FUNCTION "ROBOT_INRFACE" : VOID
TITLE =BLOCK ROBOT 1 AND 2 INTERFACE
AUTHOR : Esposito
FAMILY : EGAL_srl
NAME : ROB_INT
VERSION : 0.1


VAR_TEMP
  Tem_Cycle1_1 : BOOL ;
  Tem_cycle2_1 : BOOL ;
  Tem_cycle3_1 : BOOL ;
  Tem_cycle1_2 : BOOL ;
  Tem_cycle2_2 : BOOL ;
  Tem_cycle3_2 : BOOL ;
  Cycle_R1 : BOOL ;
  Cycle_R2 : BOOL ;
  Reserve : BYTE ;
  Reserve1 : INT ;
  Reserve2 : INT ;
  Reserve3 : INT ;
  Reserve4 : INT ;
  Rob1_Cycle : INT ;
  Rob2_Cycle : INT ;
END_VAR
BEGIN
NETWORK
TITLE =RESET ROBOT 1 AND 2 - rdiResetNood1 - rdiResetNood2
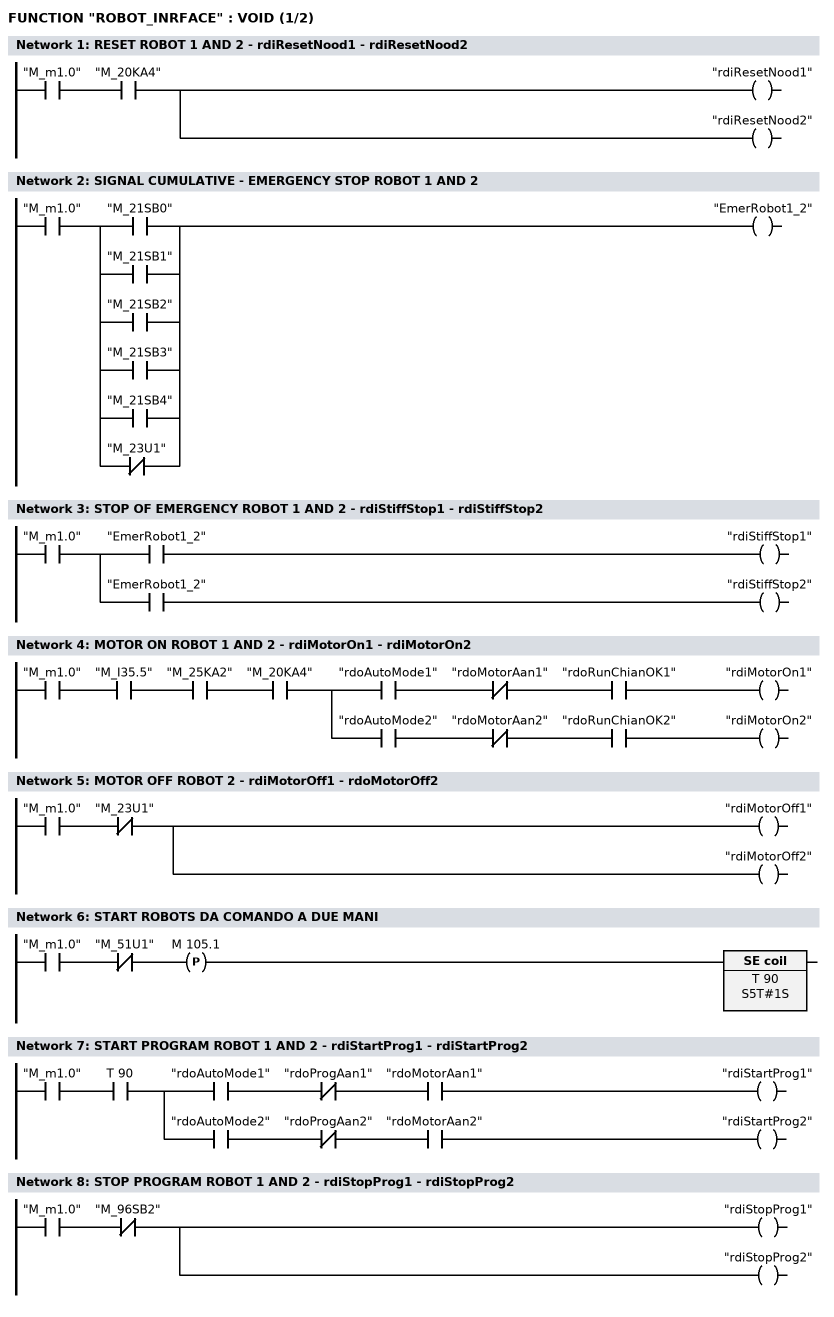
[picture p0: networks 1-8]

      U     "M_m1.0";
      U     "M_20KA4";
      =     "rdiResetNood1";
      =     "rdiResetNood2";
NETWORK
TITLE =SIGNAL CUMULATIVE - EMERGENCY STOP ROBOT 1 AND 2

      U     "M_m1.0";
      U(    ;
      O     "M_21SB0";
      O     "M_21SB1";
      O     "M_21SB2";
      O     "M_21SB3";
      O     "M_21SB4";
      ON    "M_23U1";
      )     ;
      =     "EmerRobot1_2";
NETWORK
TITLE =STOP OF EMERGENCY ROBOT 1 AND 2 - rdiStiffStop1 - rdiStiffStop2

      U     "M_m1.0";
      =     L     14.0;
      U     L     14.0;
      U     "EmerRobot1_2";
      =     "rdiStiffStop1";
      U     L     14.0;
      U     "EmerRobot1_2";
      =     "rdiStiffStop2";
NETWORK
TITLE =MOTOR ON ROBOT 1 AND 2 - rdiMotorOn1 - rdiMotorOn2

      U     "M_m1.0";
      U     "M_I35.5";
      U     "M_25KA2";
      U     "M_20KA4";
      =     L     14.0;
      U     L     14.0;
      U     "rdoAutoMode1";
      UN    "rdoMotorAan1";
      U     "rdoRunChianOK1";
      =     "rdiMotorOn1";
      U     L     14.0;
      U     "rdoAutoMode2";
      UN    "rdoMotorAan2";
      U     "rdoRunChianOK2";
      =     "rdiMotorOn2";
NETWORK
TITLE =MOTOR OFF ROBOT 2 - rdiMotorOff1 - rdoMotorOff2

      U     "M_m1.0";
      UN    "M_23U1";
      =     "rdiMotorOff1";
      =     "rdiMotorOff2";
NETWORK
TITLE =START ROBOTS DA COMANDO A DUE MANI

      U     "M_m1.0";
      UN    "M_51U1";
      FP    M    105.1;
      L     S5T#1S;
      SV    T     90;
NETWORK
TITLE =START PROGRAM ROBOT 1 AND 2 - rdiStartProg1 - rdiStartProg2

      U     "M_m1.0";
      U     T     90;
      =     L     14.0;
      U     L     14.0;
      U     "rdoAutoMode1";
      UN    "rdoProgAan1";
      U     "rdoMotorAan1";
      =     "rdiStartProg1";
      U     L     14.0;
      U     "rdoAutoMode2";
      UN    "rdoProgAan2";
      U     "rdoMotorAan2";
      =     "rdiStartProg2";
NETWORK
TITLE =STOP PROGRAM ROBOT 1 AND 2 - rdiStopProg1 - rdiStopProg2

      U     "M_m1.0";
      UN    "M_96SB2";
      =     "rdiStopProg1";
      =     "rdiStopProg2";
NETWORK
TITLE =NUMBER CYCLE ROBOT 1 - rdiCYCLE1/1, 2/1, 3/1
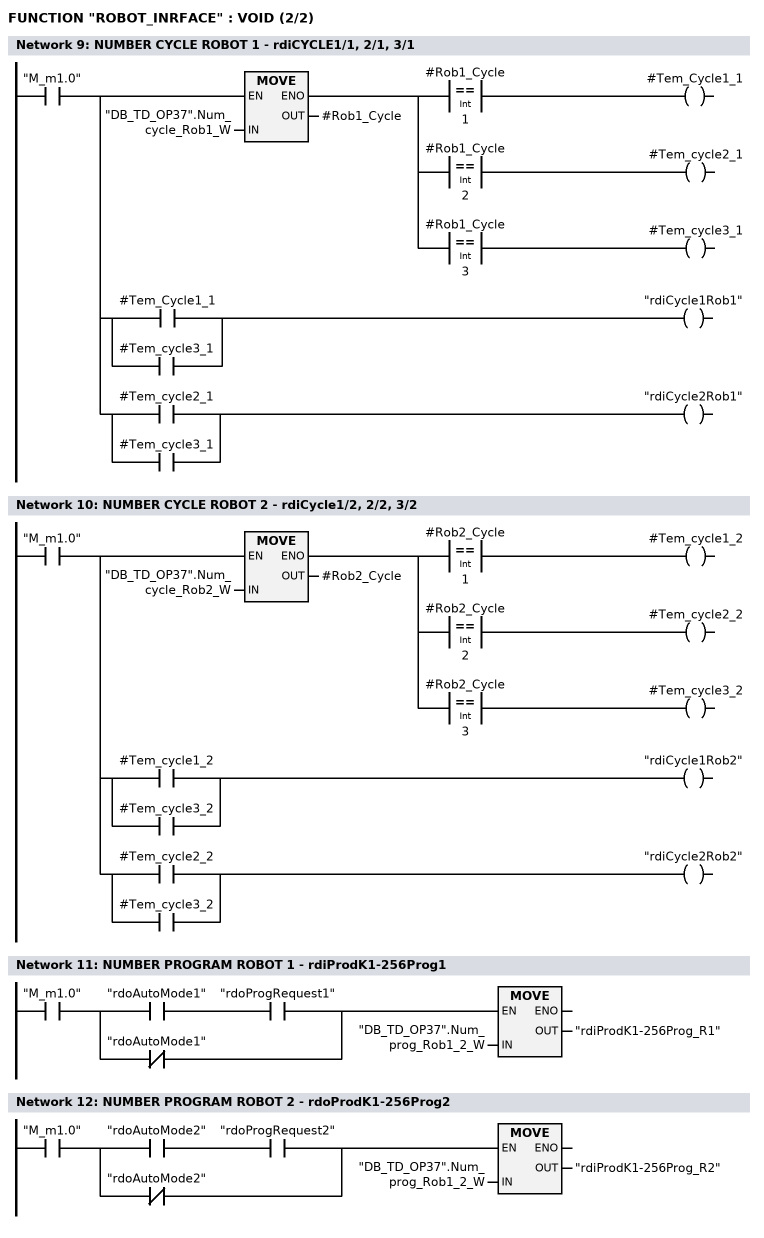
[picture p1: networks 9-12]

      U     "M_m1.0";
      =     L     14.0;
      U     L     14.0;
      SPBNB _001;
      L     "DB_TD_OP37".Num_cycle_Rob1_W;
      T     #Rob1_Cycle;
      SET   ;
      SAVE  ;
      CLR   ;
_001: U     BIE;
      =     L     14.1;
      U     L     14.1;
      U(    ;
      L     #Rob1_Cycle;
      L     1;
      ==I   ;
      )     ;
      =     #Tem_Cycle1_1;
      U     L     14.1;
      U(    ;
      L     #Rob1_Cycle;
      L     2;
      ==I   ;
      )     ;
      =     #Tem_cycle2_1;
      U     L     14.1;
      U(    ;
      L     #Rob1_Cycle;
      L     3;
      ==I   ;
      )     ;
      =     #Tem_cycle3_1;
      U     L     14.0;
      U(    ;
      O     #Tem_Cycle1_1;
      O     #Tem_cycle3_1;
      )     ;
      =     "rdiCycle1Rob1";
      U     L     14.0;
      U(    ;
      O     #Tem_cycle2_1;
      O     #Tem_cycle3_1;
      )     ;
      =     "rdiCycle2Rob1";
NETWORK
TITLE =NUMBER CYCLE ROBOT 2 - rdiCycle1/2, 2/2, 3/2



      U     "M_m1.0";
      =     L     14.0;
      U     L     14.0;
      SPBNB _002;
      L     "DB_TD_OP37".Num_cycle_Rob2_W;
      T     #Rob2_Cycle;
      SET   ;
      SAVE  ;
      CLR   ;
_002: U     BIE;
      =     L     14.1;
      U     L     14.1;
      U(    ;
      L     #Rob2_Cycle;
      L     1;
      ==I   ;
      )     ;
      =     #Tem_cycle1_2;
      U     L     14.1;
      U(    ;
      L     #Rob2_Cycle;
      L     2;
      ==I   ;
      )     ;
      =     #Tem_cycle2_2;
      U     L     14.1;
      U(    ;
      L     #Rob2_Cycle;
      L     3;
      ==I   ;
      )     ;
      =     #Tem_cycle3_2;
      U     L     14.0;
      U(    ;
      O     #Tem_cycle1_2;
      O     #Tem_cycle3_2;
      )     ;
      =     "rdiCycle1Rob2";
      U     L     14.0;
      U(    ;
      O     #Tem_cycle2_2;
      O     #Tem_cycle3_2;
      )     ;
      =     "rdiCycle2Rob2";
NETWORK
TITLE =NUMBER PROGRAM ROBOT 1 - rdiProdK1-256Prog1

      U     "M_m1.0";
      U(    ;
      U     "rdoAutoMode1";
      U     "rdoProgRequest1";
      ON    "rdoAutoMode1";
      )     ;
      SPBNB _003;
      L     "DB_TD_OP37".Num_prog_Rob1_2_W;
      T     "rdiProdK1-256Prog_R1";
_003: NOP   0;
NETWORK
TITLE =NUMBER PROGRAM ROBOT 2 - rdoProdK1-256Prog2

      U     "M_m1.0";
      U(    ;
      U     "rdoAutoMode2";
      U     "rdoProgRequest2";
      ON    "rdoAutoMode2";
      )     ;
      SPBNB _004;
      L     "DB_TD_OP37".Num_prog_Rob1_2_W;
      T     "rdiProdK1-256Prog_R2";
_004: NOP   0;
NETWORK
TITLE =CONTROL SEND PROGRAM ROBOT 1

      U     "M_m1.0";
      L     "DB_TD_OP37".Num_prog_Rob1_2_W;
      L     "rdoProdK1Prog_R1";
      ==I   ;
      =     "M_m102.6";
NETWORK
TITLE =CONTROL SEND PROGRAM ROBOT 2

      U     "M_m1.0";
      L     "DB_TD_OP37".Num_prog_Rob1_2_W;
      L     "rdoProdK1Prog_R2";
      ==I   ;
      =     "M_m102.7";
NETWORK
TITLE =PROGRAM IN JOB OK ROBOT 1 AND 2 - rdiProgNrOk1 - rdiProgNrOk2
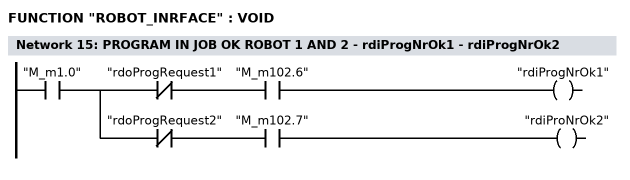
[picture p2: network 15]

      U     "M_m1.0";
      =     L     14.0;
      U     L     14.0;
      UN    "rdoProgRequest1";
      U     "M_m102.6";
      =     "rdiProgNrOk1";
      U     L     14.0;
      UN    "rdoProgRequest2";
      U     "M_m102.7";
      =     "rdiProNrOk2";
NETWORK
TITLE =ALARM ROBOT 1 - rdoRobot1Inf1-128

      U     "M_m1.0";
      L     "rdoRobot1InfB1-128";
      L     0;
      ==I   ;
      =     "M_m110.1";
NETWORK
TITLE =ALARM ROBOT 2 - rdoRobot2Inf1-128

      U     "M_m1.0";
      L     "rdoRobot2InfB1-128";
      L     0;
      ==I   ;
      =     "M_m110.0";


NETWORK
TITLE =COUNTER PARTS FROM ROBOT 2 CONTAPEZZI

      U     "M_m1.0";
      SPBNB _005;
      CALL "PACK" , DB     6 (
           TABLE                    := DB4.DBP#  50,
           P_DATA1                  := P#E 7.0 BYTE 1,
           P_DATA2                  := P#E 6.0 BYTE 1,
           ERR_CODE                 := MW    82);
_005: NOP   0;
NETWORK
TITLE =COUNTER PARTS ROBOT 1 CONTAPEZZI

      U     "M_m1.0";
      SPBNB _006;
      CALL FB    88 , DB     8 (
           TABLE                    := DB4.DBP#  56,
           P_DATA1                  := P#E 15.0 BYTE 1,
           P_DATA2                  := P#E 14.0 BYTE 1,
           ERR_CODE                 := MW    84);
_006: NOP   0;
END_FUNCTION

